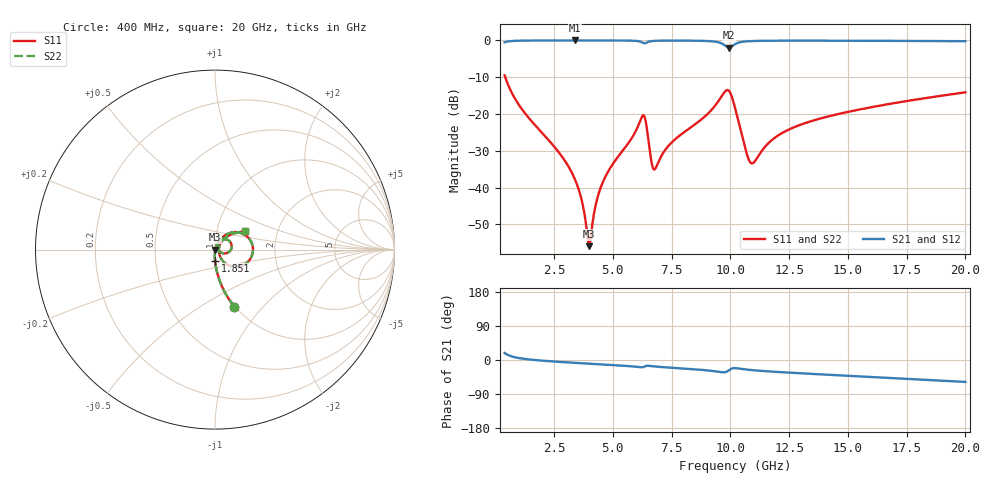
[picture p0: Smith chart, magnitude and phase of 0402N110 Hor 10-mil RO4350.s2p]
# GHz S MA R 50
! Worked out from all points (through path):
!   1960 points, 400 MHz to 20 GHz, reference 50 ohm
!   highest |S21| = -0.01 dB at 3.382 GHz (marker M1); lowest = -1.9 dB at 9.945 GHz (marker M2)
!   group delay of S21, straight-line fit = 8.58 ps
!   lowest |S11| = -55.9 dB at 3.992 GHz (marker M3), VSWR 1.00, Z = 50.2 - j0.0396 ohm
!   |S11| at or under -10 dB: 426.7 MHz to end of sweep
!   |S22| runs from -55.9 to -9.5 dB; largest |S21 - S12| = 0
!   S11 on the Smith chart (normalised r, x): 400 MHz: 0.99, -0.71; 1.851 GHz: 0.99, -0.12; 20 GHz: 1.37, +0.29
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0.4  0.3354 -71.3  0.9415 18.6  0.9415 18.6  0.3354 -71.3
0.970291  0.1388 -84.0  0.9895 5.6  0.9895 5.6  0.1388 -84.0
1.85074  0.06218 -90.0  0.9969 -0.9  0.9969 -0.9  0.06218 -90.0
3.381521  0.01318 -91.3  0.9983 -7.5  0.9983 -7.5  0.01318 -91.3
3.671669  0.006924 -86.0  0.9983 -8.5  0.9983 -8.5  0.006924 -86.0
3.991833  0.001603 -14.2  0.9982 -9.7  0.9982 -9.7  0.001603 -14.2
4.301991  0.006365 63.5  0.9981 -10.8  0.9981 -10.8  0.006365 63.5
4.582134  0.01195 69.2  0.9979 -11.8  0.9979 -11.8  0.01195 69.2
6.252986  0.0929 31.0  0.9378 -19.2  0.9378 -19.2  0.0929 31.0
6.403063  0.07898 -9.9  0.9211 -16.0  0.9211 -16.0  0.07898 -9.9
6.703216  0.01872 1.2  0.9819 -16.5  0.9819 -16.5  0.01872 1.2
6.943338  0.02234 47.8  0.9903 -17.9  0.9903 -17.9  0.02234 47.8
7.463604  0.0398 61.9  0.9935 -20.3  0.9935 -20.3  0.0398 61.9
9.51465  0.153 39.6  0.9386 -31.2  0.9386 -31.2  0.153 39.6
9.94487  0.2058 -12.2  0.7991 -26.9  0.7991 -26.9  0.2058 -12.2
10.205  0.1201 -48.1  0.8908 -21.4  0.8908 -21.4  0.1201 -48.1
10.69525  0.02922 -39.6  0.9712 -25.2  0.9712 -25.2  0.02922 -39.6
10.91536  0.02134 -3.3  0.9799 -26.6  0.9799 -26.6  0.02134 -3.3
11.9559  0.04925 49.3  0.9903 -31.4  0.9903 -31.4  0.04925 49.3
13.46667  0.08045 49.6  0.991 -36.7  0.991 -36.7  0.08045 49.6
16.73834  0.1365 40.9  0.9857 -47.3  0.9857 -47.3  0.1365 40.9
20  0.1971 30.8  0.9752 -57.9  0.9752 -57.9  0.1971 30.8
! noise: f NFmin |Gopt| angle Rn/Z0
0.4  0.001253  0.7848  1.576  0.001196
2.571  0.004661  0.6552  6.426  0.002568
4.752  0.008105  0.6386  11.43  0.00419
6.933  0.02082  0.7785  16.72  0.01884
9.104  0.03193  0.8088  21.77  0.03355
11.29  0.03069  0.7622  26.96  0.02478
13.47  0.02168  0.6324  31.55  0.01031
15.64  0.02156  0.5883  35.97  0.008722
17.82  0.02274  0.5679  40.29  0.00846
20  0.02436  0.558  44.47  0.008583
